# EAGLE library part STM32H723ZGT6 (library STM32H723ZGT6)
Arm Cortex-M7 32-bit 550 MHz MCU, up to 1 MB Flash, 564KB RAM, Ethernet, USB, 3xFD-CAN, Graphics, 2x16-bit ADCs Source: Datasheet
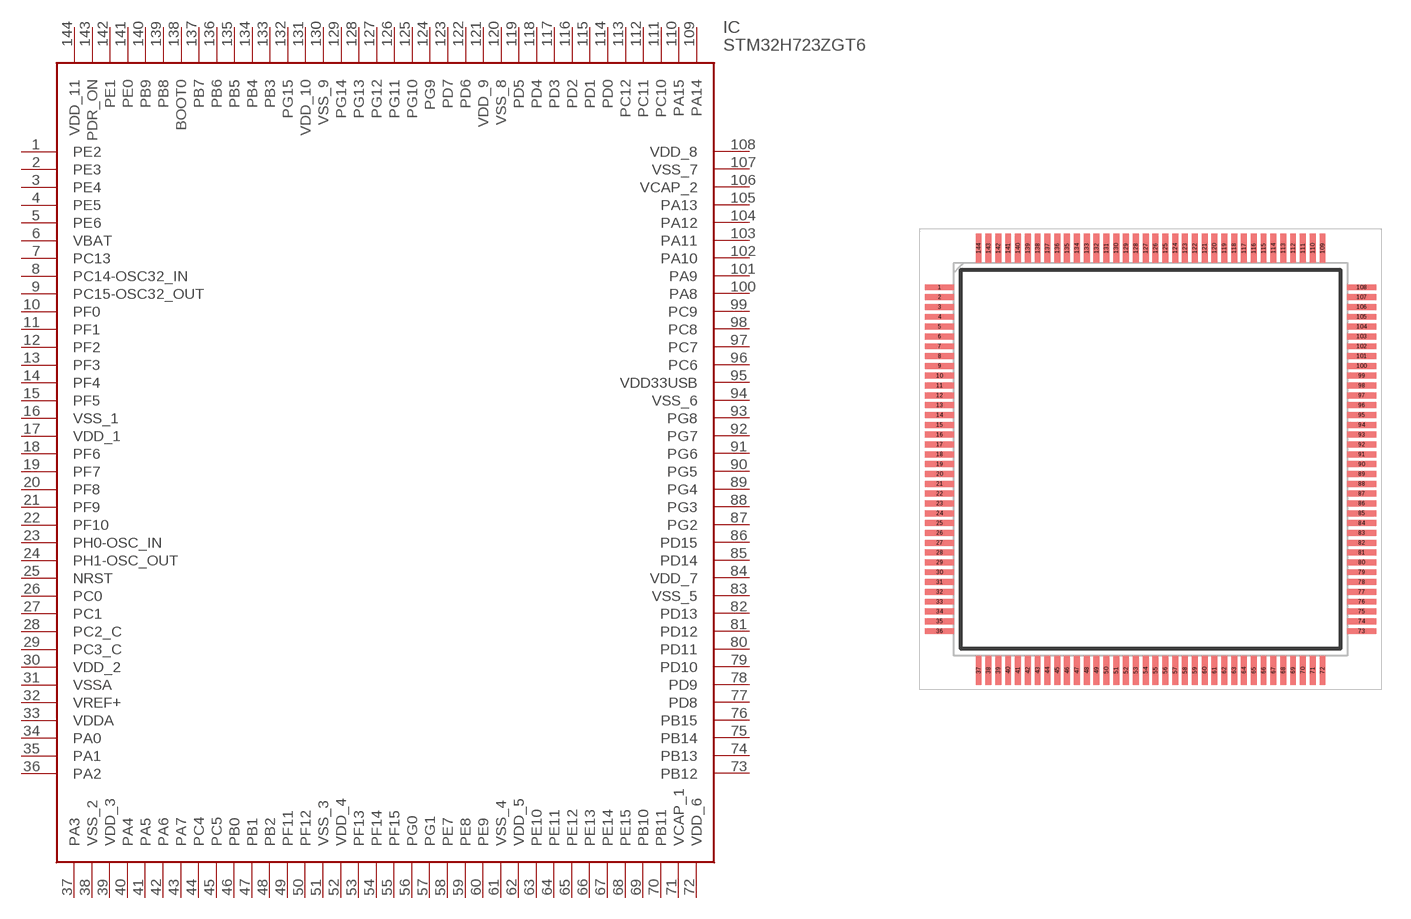
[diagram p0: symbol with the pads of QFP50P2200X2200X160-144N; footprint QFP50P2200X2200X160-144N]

Designator prefix IC

## STM32H723ZGT6 (Arrow_Part_Number: STM32H723ZGT6; Arrow_Price-Stock: https://www.arrow.com/en/products/stm32h723zgt6/stmicroelectronics?utm_currency=USD&region=nac; Description: Arm Cortex-M7 32-bit 550 MHz MCU, up to 1 MB Flash, 564KB RAM, Ethernet, USB, 3xFD-CAN, Graphics, 2x16-bit ADCs; Height: 1.6mm; Manufacturer_Name: STMicroelectronics; Manufacturer_Part_Number: STM32H723ZGT6; Mouser_Part_Number: 511-STM32H723ZGT6; Mouser_Price-Stock: https://www.mouser.co.uk/ProductDetail/STMicroelectronics/STM32H723ZGT6?qs=sPbYRqrBIVkPaOxQT7wG%252BA%3D%3D)  [QFP50P2200X2200X160-144N]
1  PE2
2  PE3
3  PE4
4  PE5
5  PE6
6  VBAT
7  PC13
8  PC14-OSC32_IN
9  PC15-OSC32_OUT
10  PF0
11  PF1
12  PF2
13  PF3
14  PF4
15  PF5
16  VSS_1
17  VDD_1
18  PF6
19  PF7
20  PF8
21  PF9
22  PF10
23  PH0-OSC_IN
24  PH1-OSC_OUT
25  NRST
26  PC0
27  PC1
28  PC2_C
29  PC3_C
30  VDD_2
31  VSSA
32  VREF+
33  VDDA
34  PA0
35  PA1
36  PA2
37  PA3
38  VSS_2
39  VDD_3
40  PA4
41  PA5
42  PA6
43  PA7
44  PC4
45  PC5
46  PB0
47  PB1
48  PB2
49  PF11
50  PF12
51  VSS_3
52  VDD_4
53  PF13
54  PF14
55  PF15
56  PG0
57  PG1
58  PE7
59  PE8
60  PE9
61  VSS_4
62  VDD_5
63  PE10
64  PE11
65  PE12
66  PE13
67  PE14
68  PE15
69  PB10
70  PB11
71  VCAP_1
72  VDD_6
73  PB12
74  PB13
75  PB14
76  PB15
77  PD8
78  PD9
79  PD10
80  PD11
81  PD12
82  PD13
83  VSS_5
84  VDD_7
85  PD14
86  PD15
87  PG2
88  PG3
89  PG4
90  PG5
91  PG6
92  PG7
93  PG8
94  VSS_6
95  VDD33USB
96  PC6
97  PC7
98  PC8
99  PC9
100  PA8
101  PA9
102  PA10
103  PA11
104  PA12
105  PA13
106  VCAP_2
107  VSS_7
108  VDD_8
109  PA14
110  PA15
111  PC10
112  PC11
113  PC12
114  PD0
115  PD1
116  PD2
117  PD3
118  PD4
119  PD5
120  VSS_8
121  VDD_9
122  PD6
123  PD7
124  PG9
125  PG10
126  PG11
127  PG12
128  PG13
129  PG14
130  VSS_9
131  VDD_10
132  PG15
133  PB3
134  PB4
135  PB5
136  PB6
137  PB7
138  BOOT0
139  PB8
140  PB9
141  PE0
142  PE1
143  PDR_ON
144  VDD_11

## Footprint QFP50P2200X2200X160-144N (pad centres in mm)
LQFP144_
smd 1.475 x 0.3: 1 -10.738,8.75; 2 -10.738,8.25; 3 -10.738,7.75; 4 -10.738,7.25; 5 -10.738,6.75; 6 -10.738,6.25; 7 -10.738,5.75; 8 -10.738,5.25; 9 -10.738,4.75; 10 -10.738,4.25; 11 -10.738,3.75; 12 -10.738,3.25; 13 -10.738,2.75; 14 -10.738,2.25; 15 -10.738,1.75; 16 -10.738,1.25; 17 -10.738,0.75; 18 -10.738,0.25; 19 -10.738,-0.25; 20 -10.738,-0.75; 21 -10.738,-1.25; 22 -10.738,-1.75; 23 -10.738,-2.25; 24 -10.738,-2.75; 25 -10.738,-3.25; 26 -10.738,-3.75; 27 -10.738,-4.25; 28 -10.738,-4.75; 29 -10.738,-5.25; 30 -10.738,-5.75; 31 -10.738,-6.25; 32 -10.738,-6.75; 33 -10.738,-7.25; 34 -10.738,-7.75; 35 -10.738,-8.25; 36 -10.738,-8.75; 73 10.738,-8.75; 74 10.738,-8.25; 75 10.738,-7.75; 76 10.738,-7.25; 77 10.738,-6.75; 78 10.738,-6.25; 79 10.738,-5.75; 80 10.738,-5.25; 81 10.738,-4.75; 82 10.738,-4.25; 83 10.738,-3.75; 84 10.738,-3.25; 85 10.738,-2.75; 86 10.738,-2.25; 87 10.738,-1.75; 88 10.738,-1.25; 89 10.738,-0.75; 90 10.738,-0.25; 91 10.738,0.25; 92 10.738,0.75; 93 10.738,1.25; 94 10.738,1.75; 95 10.738,2.25; 96 10.738,2.75; 97 10.738,3.25; 98 10.738,3.75; 99 10.738,4.25; 100 10.738,4.75; 101 10.738,5.25; 102 10.738,5.75; 103 10.738,6.25; 104 10.738,6.75; 105 10.738,7.25; 106 10.738,7.75; 107 10.738,8.25; 108 10.738,8.75
smd 0.3 x 1.475: 37 -8.75,-10.738; 38 -8.25,-10.738; 39 -7.75,-10.738; 40 -7.25,-10.738; 41 -6.75,-10.738; 42 -6.25,-10.738; 43 -5.75,-10.738; 44 -5.25,-10.738; 45 -4.75,-10.738; 46 -4.25,-10.738; 47 -3.75,-10.738; 48 -3.25,-10.738; 49 -2.75,-10.738; 50 -2.25,-10.738; 51 -1.75,-10.738; 52 -1.25,-10.738; 53 -0.75,-10.738; 54 -0.25,-10.738; 55 0.25,-10.738; 56 0.75,-10.738; 57 1.25,-10.738; 58 1.75,-10.738; 59 2.25,-10.738; 60 2.75,-10.738; 61 3.25,-10.738; 62 3.75,-10.738; 63 4.25,-10.738; 64 4.75,-10.738; 65 5.25,-10.738; 66 5.75,-10.738; 67 6.25,-10.738; 68 6.75,-10.738; 69 7.25,-10.738; 70 7.75,-10.738; 71 8.25,-10.738; 72 8.75,-10.738; 109 8.75,10.738; 110 8.25,10.738; 111 7.75,10.738; 112 7.25,10.738; 113 6.75,10.738; 114 6.25,10.738; 115 5.75,10.738; 116 5.25,10.738; 117 4.75,10.738; 118 4.25,10.738; 119 3.75,10.738; 120 3.25,10.738; 121 2.75,10.738; 122 2.25,10.738; 123 1.75,10.738; 124 1.25,10.738; 125 0.75,10.738; 126 0.25,10.738; 127 -0.25,10.738; 128 -0.75,10.738; 129 -1.25,10.738; 130 -1.75,10.738; 131 -2.25,10.738; 132 -2.75,10.738; 133 -3.25,10.738; 134 -3.75,10.738; 135 -4.25,10.738; 136 -4.75,10.738; 137 -5.25,10.738; 138 -5.75,10.738; 139 -6.25,10.738; 140 -6.75,10.738; 141 -7.25,10.738; 142 -7.75,10.738; 143 -8.25,10.738; 144 -8.75,10.738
